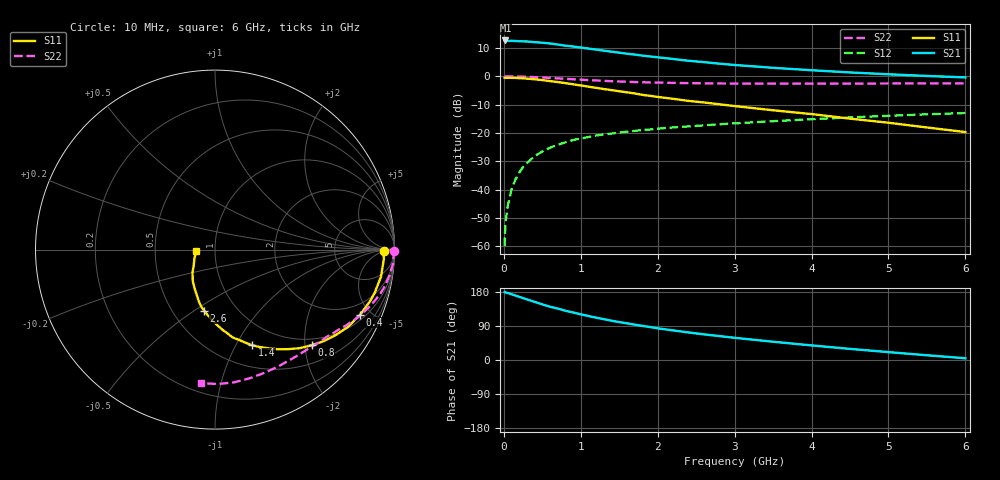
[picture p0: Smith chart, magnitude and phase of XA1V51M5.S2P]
! SIEMENS Discrete & RF Semiconductors
! BFY180
! Si NPN RF Bipolar Junction Transistor in MICRO-X
! VCE = 1.5 V  IC = 1.5 mA
! Common Emitter S-Parameters:  May  1997
# GHz  S  MA  R  50
!  f  S11  S21  S12  S22
! GHz  MAG  ANG  MAG  ANG  MAG  ANG  MAG  ANG
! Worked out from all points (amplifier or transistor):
!   36 points, 10 MHz to 6 GHz, reference 50 ohm
!   highest |S21| = 12.7 dB at 20 MHz (marker M1)
!   |S21| within 3 dB of that: start of sweep to 1.137 GHz
!   unconditionally stable (mu >= 1): 2.749 GHz to end of sweep
!   at 250 MHz: K = 0.12, MSG = 22.2 dB, |S12| = -32.0 dB
!   at 1.4 GHz: K = 0.67, MSG = 14.5 dB, |S12| = -20.2 dB
!   at 6 GHz: K = 1.10, MAG = 4.4 dB, |S12| = -13.0 dB
!   S11 on the Smith chart (normalised r, x): 10 MHz: 32, -5; 400 MHz: 1.28, -4.32; 800 MHz: 0.86, -2.14; 1.4 GHz: 0.74, -1.16; 2.6 GHz: 0.71, -0.55; 6 GHz: 0.81, -0.01
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0.01  0.941 -0.5  4.231 179.5  0.001 82.7  0.997 -0.3
0.02  0.9387 -1.2  4.297 178.6  0.0025 90.3  0.9998 -0.7
0.05  0.9423 -3.1  4.21 176.8  0.0051 87.5  0.9958 -1.6
0.1  0.9383 -6.1  4.238 173.5  0.0101 86.9  0.9953 -3.2
0.15  0.9369 -9.3  4.203 170.0  0.015 82.8  0.9934 -4.8
0.3  0.9104 -18.4  4.126 159.8  0.0294 78.1  0.9782 -9.4
0.4  0.8864 -24.1  4.004 153.4  0.0389 74.4  0.9677 -12.2
0.5  0.8566 -30.2  3.92 146.9  0.047 70.8  0.953 -15.0
0.6  0.8234 -35.4  3.802 140.5  0.0547 67.2  0.9361 -17.5
0.8  0.7574 -44.7  3.475 130.0  0.0682 61.2  0.9025 -22.3
1  0.6889 -53.6  3.228 120.4  0.08 56.3  0.8731 -26.3
1.1  0.6567 -57.7  3.087 116.1  0.0847 54.5  0.8579 -28.0
1.4  0.5709 -68.9  2.722 103.7  0.0976 49.2  0.8194 -33.1
1.8  0.4698 -81.8  2.321 90.1  0.1124 44.5  0.7865 -39.0
2  0.4321 -86.8  2.167 83.6  0.1189 42.4  0.7751 -41.8
2.2  0.4004 -91.2  2.023 78.1  0.1251 40.4  0.7655 -44.6
2.6  0.345 -100.3  1.781 67.7  0.1361 37.5  0.7515 -49.8
3  0.2982 -107.9  1.585 58.6  0.1475 34.4  0.7441 -54.9
3.5  0.2512 -116.2  1.413 48.2  0.1612 31.0  0.7402 -61.3
4.5  0.1788 -134.6  1.17 29.3  0.1879 23.8  0.7424 -74.6
5.5  0.1248 -156.9  1.014 12.5  0.2133 15.9  0.7492 -88.8
6  0.1036 -175.2  0.956 4.6  0.2247 11.6  0.7483 -96.0
